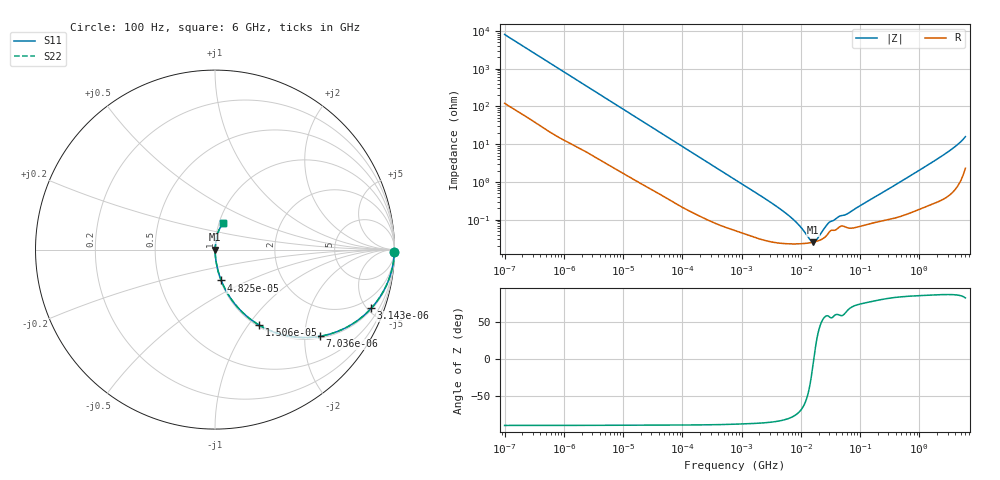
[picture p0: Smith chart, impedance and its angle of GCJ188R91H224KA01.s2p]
!Murata Part Number: GCJ188R91H224KA01
!These Parameters are Measured in Series Mode Connection
!Data Generated on Mar 13, 2026
!  o--ll--o
!Port1  Port2
!  o------o
!Operation Temp=25[degC], DC Bias Voltage=0[V]
!Freq. Start=100[Hz] Stop=6[GHz] 401[Steps]
# Hz S RI R 50
!Freq.(Hz) S11(Real) S11(Imag) S21(Real) S21(Imag) S12(Real) S12(Imag) S22(Real) S22(Imag)
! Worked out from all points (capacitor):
!   401 points, 100 Hz to 6 GHz, reference 50 ohm
!   read as one part in series: C = 197 nF near 109 Hz
!   lowest |Z| = 25.5 mohm at 16.27 MHz (marker M1)
!   series resonance near 16.57 MHz, so ESL is about 470 pH
!   S11 on the Smith chart (normalised r, x): 100 Hz: open; 3.143 kHz: 1.10, -5.29; 7.036 kHz: 1.05, -2.39; 15.06 kHz: 1.02, -1.12; 48.25 kHz: 1.01, -0.36; 6 GHz: 1.05, +0.31
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100  0.9997 -0.0124  0.000343 0.0124  0.000343 0.0124  0.9997 -0.0124
600  0.9936 -0.0728  0.00642 0.0728  0.00642 0.0728  0.9936 -0.0728
2008  0.9407 -0.2275  0.0593 0.2275  0.0593 0.2275  0.9407 -0.2275
3143  0.8704 -0.3268  0.1296 0.3268  0.1296 0.3268  0.8704 -0.3268
7036  0.5856 -0.483  0.4144 0.483  0.4144 0.483  0.5856 -0.483
15062  0.2449 -0.4198  0.7551 0.4198  0.7551 0.4198  0.2449 -0.4198
23569  0.1209 -0.3154  0.8791 0.3154  0.8791 0.3154  0.1209 -0.3154
40335  0.0476 -0.2018  0.9524 0.2018  0.9524 0.2018  0.0476 -0.2018
48246  0.0346 -0.1716  0.9654 0.1716  0.9654 0.1716  0.0346 -0.1716
147774  0.00501 -0.0588  0.995 0.0588  0.995 0.0588  0.00501 -0.0588
774597  0.000648 -0.0115  0.9994 0.0115  0.9994 0.0115  0.000648 -0.0115
5809218  0.000233 -0.0014  0.9998 0.0014  0.9998 0.0014  0.000233 -0.0014
9090158  0.00023 -0.000714  0.9998 0.000714  0.9998 0.000714  0.00023 -0.000714
1.555665e7  0.00025 -7.14e-05  0.9997 7.14e-05  0.9997 7.14e-05  0.00025 -7.14e-05
1.626902e7  0.000254 -2.08e-05  0.9997 2.08e-05  0.9997 2.08e-05  0.000254 -2.08e-05
1.86079e7  0.000268 0.000132  0.9997 -0.000132  0.9997 -0.000132  0.000268 0.000132
3.045065e7  0.000478 0.000717  0.9995 -0.000717  0.9995 -0.000717  0.000478 0.000717
4.35672e7  0.000619 0.00103  0.9994 -0.00103  0.9994 -0.00103  0.000619 0.00103
6.233367e7  0.000608 0.00133  0.9994 -0.00133  0.9994 -0.00133  0.000608 0.00133
3.124326e8  0.00106 0.00661  0.9989 -0.00661  0.9989 -0.00661  0.00106 0.00661
2.450438e9  0.00577 0.049  0.9942 -0.049  0.9942 -0.049  0.00577 0.049
6e9  0.0449 0.1461  0.9551 -0.1461  0.9551 -0.1461  0.0449 0.1461
